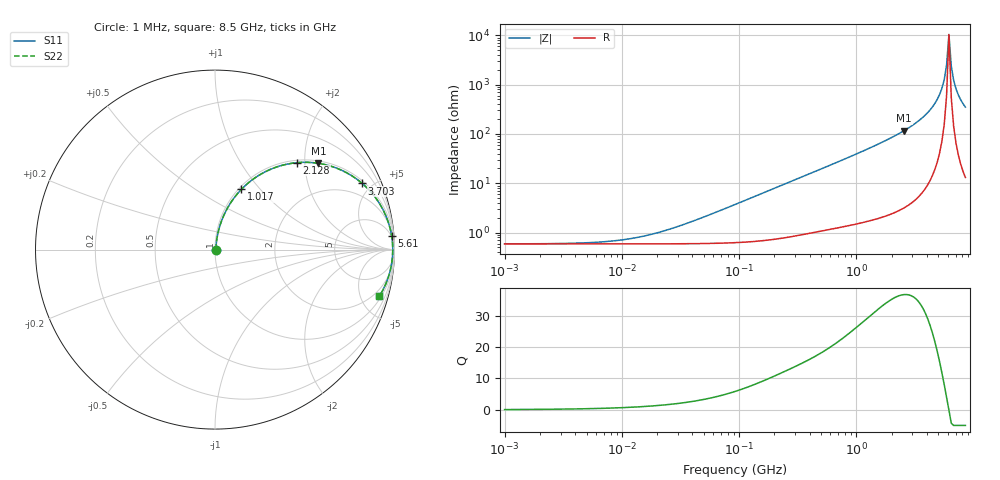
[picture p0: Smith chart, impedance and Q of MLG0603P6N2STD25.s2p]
! S-Parameter Data Generated by TDK Corporation
! Copyright(C) 2025 TDK Corporation.
! All Rights Reserved.
! TDK P/N: MLG0603P6N2STD25 (SMD / SMT Inductor (Coil))
! Property: L=6.2nH at 500MHz
! Size(LxWxT): 0.6x0.3x0.3mm
! Model Type: s2p (Touchstone File Format Version 1.0)
! Frequency: DC=Yes Start=1MHz Stop=8500MHz 198points Log-sweep
! Model Generated on Feb. 6, 2025
! Terms and conditions regarding TDK Simulation Models:
! 1)This simulation model is being provided solely for informational
!  purposes. Please refer to the specifications of the products in
!  terms of detailed characteristics of such products.
! 2)In no event shall TDK Corporation of any of its subsidiaries be
!  liable for any loss or damage arising, directly or indirectly,
!  from any information contained in this simulation model, including,
!  but not limited to loss or damages arising from any inaccuracies,
!  omissions or errors in connection with such information.
! 3)Any and all copyrights on this simulation model are owned by
!  TDK Corporation.  Duplication or redistribution of this simulation
!  model without prior written permission from TDK Corporation
!  is prohibited.
! 4)This simulation model is subject to any modification or change
!  without any prior notice.
! 5)Neither TDK Corporation nor any of its subsidiaries shall make any
!  warranty, express or implied, including but not limited to the
!  correctness, implied warranties of merchantability and fitness for
!  a particular purpose with respect to this simulation models.
! 6)The use of this simulation model shall be deemed to have consented
!  to the terms and conditions hereof.
! Port Assignments:
!  1 ---@@@--- 2
! Applicable Conditions:
!  Temperature = 25 degC
!  DC Bias Current = 0 A
!  Small Signal Operation
# Hz S MA R 50
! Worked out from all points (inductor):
!   197 points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, 1 MHz to 8.5 GHz, reference 50 ohm
!   read as one part in series: L = 6.31 nH near 46.13 MHz
!   highest Q = 36.8 at 2.56 GHz (marker M1), where L = 7.28 nH
!   self-resonance near 5.875 GHz
!   S11 on the Smith chart (normalised r, x): 1 MHz: 1.01, +0.00; 1.017 GHz: 1.03, +0.80; 2.128 GHz: 1.05, +1.83; 3.703 GHz: 1.14, +4.38; 5.61 GHz: 4, +25; 8.5 GHz: 1.26, -6.99
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1000000  0.005879 3.8  0.9941 -0.0  0.9941 -0.0  0.005879 3.8
4587603  0.006139 17.1  0.9941 -0.1  0.9941 -0.1  0.006139 17.1
1.053054e7  0.007193 35.1  0.9941 -0.2  0.9941 -0.2  0.007193 35.1
2.10461e7  0.01018 54.2  0.9941 -0.5  0.9941 -0.5  0.01018 54.2
9.219544e7  0.03682 78.2  0.9931 -2.1  0.9931 -2.1  0.03682 78.2
4.229561e8  0.1616 77.3  0.9772 -9.3  0.9772 -9.3  0.1616 77.3
1.016736e9  0.3664 66.4  0.9168 -21.5  0.9168 -21.5  0.3664 66.4
1.404574e9  0.4846 59.2  0.8592 -29.0  0.8592 -29.0  0.4846 59.2
1.940355e9  0.6241 49.8  0.7637 -38.6  0.7637 -38.6  0.6241 49.8
2.128028e9  0.6662 46.6  0.7274 -41.8  0.7274 -41.8  0.6662 46.6
2.559585e9  0.7505 39.8  0.6408 -48.6  0.6408 -48.6  0.7505 39.8
3.703002e9  0.8994 24.2  0.4103 -64.0  0.4103 -64.0  0.8994 24.2
4.253027e9  0.9407 17.8  0.306 -70.1  0.306 -70.1  0.9407 17.8
4.884749e9  0.9706 11.2  0.1945 -75.7  0.1945 -75.7  0.9706 11.2
5.357206e9  0.9832 6.7  0.1175 -78.4  0.1175 -78.4  0.9832 6.7
5.610304e9  0.9872 4.5  0.0785 -78.4  0.0785 -78.4  0.9872 4.5
5.87536e9  0.9897 2.2  0.03967 -73.8  0.03967 -73.8  0.9897 2.2
6.152938e9  0.9905 -0.1  0.00955 6.1  0.00955 6.1  0.9905 -0.1
6.44363e9  0.9897 -2.3  0.04164 74.6  0.04164 74.6  0.9897 -2.3
6.748056e9  0.9873 -4.6  0.08056 78.7  0.08056 78.7  0.9873 -4.6
7.400733e9  0.9778 -9.1  0.1585 77.4  0.1585 77.4  0.9778 -9.1
8.5e9  0.9521 -15.8  0.2722 72.1  0.2722 72.1  0.9521 -15.8
